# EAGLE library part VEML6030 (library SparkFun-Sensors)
VEML6030 Ambient Light Sensor VEML6030 is a high accuracy ambient light digital 16-bit resolution sensor in a miniature transparent 2 mm x 2 mm package. It includes a high sensitive photodiode, a low noise amplifier, a 16-bit A/D converter and supports an easy to use I2C bus communication interface and additional interrupt feature.
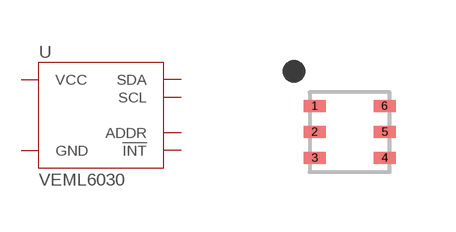
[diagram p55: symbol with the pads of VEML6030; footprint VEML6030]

Designator prefix U

## VEML6030 (PROD_ID: IC-14447)  [VEML6030]
1  GND  pwr
2  SDA
3  !INT  out
4  ADDR
5  SCL
6  VCC  pwr

## Footprint VEML6030 (pad centres in mm)
VEML6030 Ambient Light Sensor Physical Characteristics 6 Pin SMD Package 2mm x 2mm x .83mm .65mm Pitch .45mm x .4mm Pad Size
smd 0.55 x 0.3: 1 -0.88,0.65; 2 -0.88,0; 3 -0.88,-0.65; 4 0.87,-0.65; 5 0.87,0; 6 0.87,0.65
